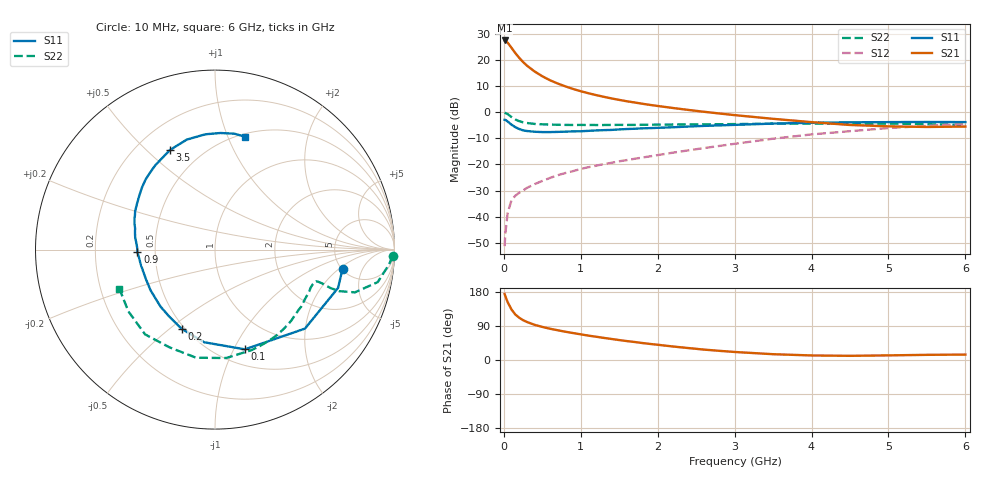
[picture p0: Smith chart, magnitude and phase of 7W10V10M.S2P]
! Infineon Technologies  Discrete & RF Semiconductors
! BFS17W
! Si NPN RF Bipolar Junction Transistor in SOT323
! VCE = 10 V  IC = 10 mA
! Common Emitter S-Parameters:  August  1999
# GHz  S  MA  R  50
!  f  S11  S21  S12  S22
! GHz  MAG  ANG  MAG  ANG  MAG  ANG  MAG  ANG
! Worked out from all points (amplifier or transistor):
!   36 points, 10 MHz to 6 GHz, reference 50 ohm
!   highest |S21| = 27.6 dB at 10 MHz (marker M1)
!   |S21| within 3 dB of that: start of sweep to 103.9 MHz
!   unconditionally stable (mu >= 1): 442.7 MHz to 2.136 GHz; 5.598 GHz to end of sweep
!   at 250 MHz: K = 0.78, MSG = 24.7 dB, |S12| = -30.0 dB
!   at 1.4 GHz: K = 1.16, MAG = 9.9 dB, |S12| = -19.4 dB
!   at 6 GHz: K = 1.03, MAG = -1.5 dB, |S12| = -4.5 dB
!   S11 on the Smith chart (normalised r, x): 10 MHz: 5.09, -2.24; 100 MHz: 0.66, -1.11; 200 MHz: 0.48, -0.55; 900 MHz: 0.40, -0.01; 3.5 GHz: 0.34, +0.59; 6 GHz: 0.53, +1.16
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0.01  0.7188 -8.5  24.04 174.1  0.0027 78.5  0.9909 -2.1
0.02  0.7181 -17.3  23.77 168.2  0.0048 85.1  0.9722 -5.0
0.05  0.667 -41.3  21.73 152.4  0.0118 73.7  0.9246 -11.3
0.1  0.5801 -73.3  17.32 133.1  0.0207 61.5  0.8151 -17.0
0.15  0.5197 -96.7  13.72 119.9  0.0252 56.8  0.7292 -18.5
0.2  0.4789 -112.8  11.14 111.5  0.0287 57.0  0.6782 -18.4
0.25  0.4512 -124.8  9.265 105.1  0.0317 55.5  0.645 -17.9
0.3  0.439 -133.9  7.904 100.4  0.0355 57.4  0.6256 -17.5
0.4  0.4246 -147.8  6.095 92.8  0.0419 59.3  0.6006 -17.3
0.5  0.4186 -156.8  4.939 87.3  0.0483 62.3  0.5898 -17.5
0.6  0.4184 -163.5  4.14 82.5  0.0551 63.6  0.5827 -18.2
0.7  0.4221 -169.1  3.583 78.5  0.0621 65.0  0.5785 -19.3
0.9  0.4324 -178.1  2.816 71.1  0.0745 66.9  0.5733 -22.1
1.1  0.4421 174.2  2.33 64.3  0.0886 68.4  0.5734 -25.6
1.3  0.4562 167.8  1.99 58.3  0.1018 69.5  0.5723 -29.5
1.6  0.4794 159.4  1.633 49.9  0.1214 70.9  0.5743 -35.6
2.2  0.5183 144.4  1.213 35.6  0.1686 73.2  0.5852 -49.6
2.8  0.562 129.9  0.953 24.2  0.2266 72.9  0.5927 -65.1
3.5  0.6092 114.3  0.752 15.3  0.3122 69.2  0.6072 -84.1
4.5  0.6446 94.8  0.573 11.0  0.4357 57.5  0.6007 -114.9
5.5  0.6548 80.5  0.525 13.6  0.5503 44.3  0.5928 -144.5
6  0.6506 75.0  0.534 14.3  0.5961 37.6  0.5755 -157.8
